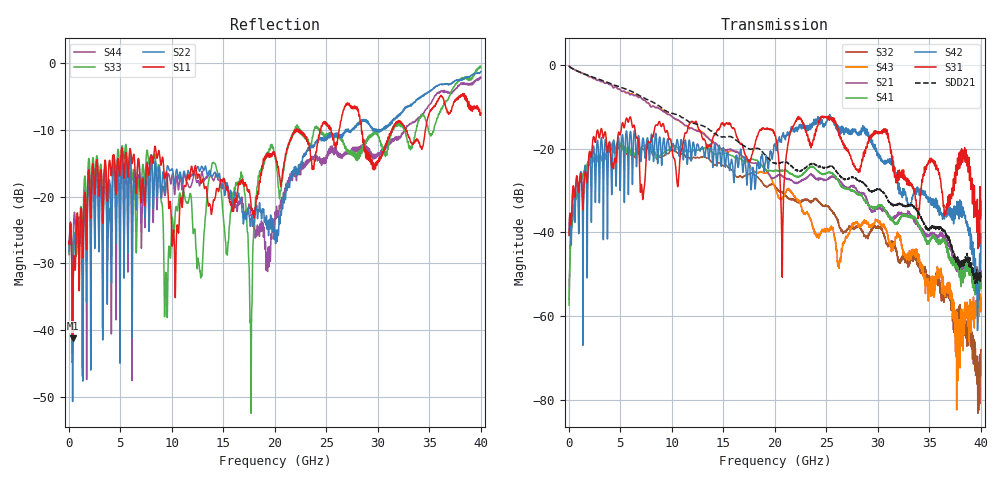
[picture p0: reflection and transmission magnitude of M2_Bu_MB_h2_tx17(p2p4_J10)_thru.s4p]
! S11 = S11
! S12 = S12
! S13 = S13
! S14 = S14
! S21 = S21
! S22 = S22
! S23 = S23
! S24 = S24
! S31 = S31
! S32 = S32
! S33 = S33
! S34 = S34
! S41 = S41
! S42 = S42
! S43 = S43
! S44 = S44
! FILE: \\englab.brocade.com\shares\Groups\SIT\Work\Shaohua\IEEE_channels\M2_Bu_MB_h2_tx17(p2p4_J10)_thru.s4p
!$DUT_CFG_DESC: Default 4-Port Configuration
!$NUMBER_PORTS: 4
!$DIFF_PORT_MAP: 1|2P|2|2P|0|UC|0|UC|
!$PORT_MAP: PNA 1|1|<<<<<<|TS 2|2|>>>>>>|PNA 2|3|<<<<<<|TS 4|4|>>>>>>|
# MHz S RI R 50.00
! FREQ  S11  S12  S13  S14
!  S21  S22  S23  S24
!  S31  S32  S33  S34
!  S41  S42  S43  S44
!  REAL  IMAG  REAL  IMAG  REAL  IMAG  REAL  IMAG
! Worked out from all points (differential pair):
!   3996 points, 50 MHz to 40 GHz, reference 50 ohm
!   strongest paths, dB at 50 MHz, 10.04 GHz, 20.03 GHz, 30.02 GHz, 40 GHz:
!     S31: -40.7, -20.2, -16.9, -16.3, -32.5
!     S42: -40.8, -19.1, -19.1, -21.3, -40.4
!     S41: -57.5, -19.4, -25.2, -33.8, -51.4
!     S21: -0.3, -12.4, -26.8, -34.1, -49.6
!     S43: -0.3, -12.4, -29.4, -37.3, -56.5
!     S32: -56.1, -20.4, -28.9, -38.5, -68.1
!   taken as a pair (ports 1,3 in; 2,4 out), SDD21 dB: -0.3, -11.6, -23.5, -29.7, -49.6
!   lowest |S11| = -41.2 dB at 380 MHz (marker M1), VSWR 1.02, Z = 50.9 + j0.113 ohm
!   |S11| at or under -10 dB: start of sweep to 21.97 GHz; 22.37 GHz to 24.46 GHz (2.09 GHz wide, 8.93 % of centre); 28.41 GHz to 31.37 GHz (2.962 GHz wide, 9.91 % of centre)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
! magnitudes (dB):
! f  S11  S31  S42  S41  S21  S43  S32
! 50 MHz  -26.9  -40.7  -40.8  -57.5  -0.3  -0.3  -56.1
! 380 MHz  -41.2  -30.4  -31.3  -37.4  -0.9  -0.9  -37.2
! 14.09 GHz  -20.6  -17.0  -21.0  -21.3  -18.5  -18.8  -23.9
! 17.66 GHz  -20.4  -22.5  -28.4  -22.8  -23.3  -24.4  -25.9
! 20.72 GHz  -17.1  -50.4  -16.9  -25.3  -26.6  -31.9  -30.4
! 25.4 GHz  -9.8  -12.8  -12.8  -25.8  -26.9  -39.3  -34.5
! 40 GHz  -7.5  -32.5  -40.4  -51.4  -49.6  -56.5  -68.1
